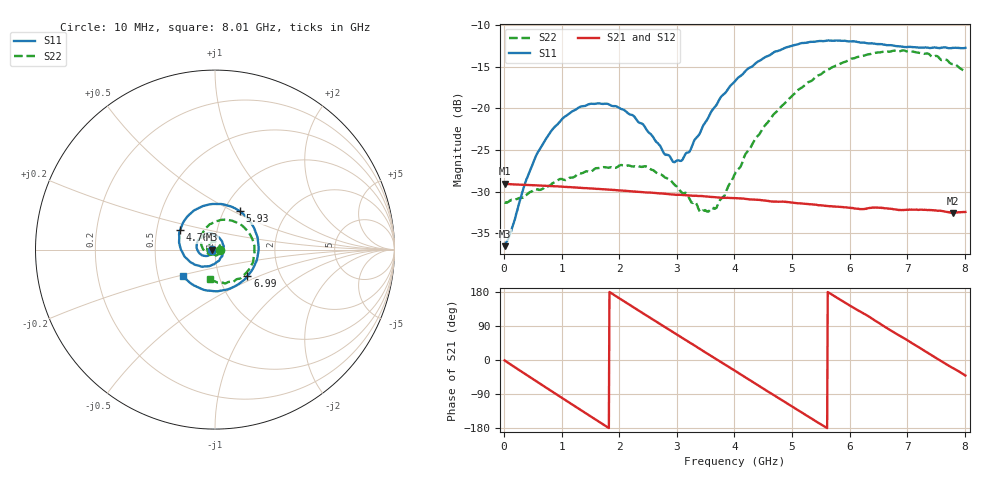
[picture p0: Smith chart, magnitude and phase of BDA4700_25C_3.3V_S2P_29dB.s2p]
!Agilent Technologies,E5071B,MY42404982,A.09.10
!Date: Mon Oct 20 18:15:16 2025
!Data & Calibration Information:
!Freq	S11:SOLT2(ON)	S21:SOLT2(ON)	S12:SOLT2(ON)	S22:SOLT2(ON)
# Hz S RI R 50
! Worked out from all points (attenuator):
!   801 points, 10 MHz to 8.01 GHz, reference 50 ohm
!   highest |S21| = -29.05 dB at 20 MHz (marker M1); lowest = -32.6 dB at 7.8 GHz (marker M2)
!   lowest |S11| = -36.5 dB at 10 MHz (marker M3), VSWR 1.03, Z = 48.5 - j0.123 ohm
!   |S11| at or under -10 dB: start of sweep to end of sweep
!   |S22| runs from -32.5 to -13.0 dB; largest |S21 - S12| = 0.00038
!   S11 on the Smith chart (normalised r, x): 10 MHz: 0.97, -0.00; 4.76 GHz: 0.66, +0.15; 5.93 GHz: 1.19, +0.54; 6.99 GHz: 1.36, -0.43; 8.01 GHz: 0.67, -0.21
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1e7  -0.0148 -0.00126  0.0352 -0.000725  0.0352 -0.000801  0.0272 -0.000793
2e7  -0.0152 -0.00199  0.0352 -0.00132  0.0352 -0.00144  0.0271 -0.00111
5.9e8  -0.042 -0.0353  0.0178 -0.0296  0.0178 -0.0295  0.0139 -0.0295
1e9  -0.0822 -0.0243  -0.00551 -0.0334  -0.00552 -0.0334  -0.0146 -0.0348
1.35e9  -0.1024 0.0116  -0.023 -0.0241  -0.023 -0.0241  -0.0364 -0.0182
2.07e9  -0.046 0.087  -0.0294 0.0129  -0.0293 0.0129  -0.0309 0.0332
2.68e9  0.0378 0.0483  -0.00406 0.0307  -0.00411 0.0306  0.0127 0.0384
2.93e9  0.0475 0.00681  0.00845 0.0292  0.00849 0.0291  0.0249 0.0256
3.06e9  0.0454 -0.0167  0.0145 0.0266  0.0142 0.0266  0.0279 0.0156
3.43e9  0.00301 -0.0752  0.0267 0.0132  0.0267 0.0133  0.0202 -0.0127
3.69e9  -0.0491 -0.0932  0.0292 0.00094  0.0293 0.000862  0.00162 -0.0253
4.01e9  -0.1237 -0.0776  0.0254 -0.0138  0.0254 -0.0137  -0.0309 -0.0261
4.41e9  -0.1915 0.00402  0.0112 -0.0259  0.0113 -0.026  -0.0683 0.00643
4.76e9  -0.1945 0.1076  -0.00461 -0.0271  -0.00451 -0.0271  -0.0783 0.0591
5.35e9  -0.0624 0.2435  -0.0241 -0.011  -0.0241 -0.0111  -0.0161 0.1465
5.93e9  0.1391 0.2134  -0.0222 0.0126  -0.0222 0.0124  0.114 0.1535
6.35e9  0.2304 0.0865  -0.01 0.0232  -0.00988 0.0231  0.1942 0.0854
6.68e9  0.2366 -0.0412  0.00386 0.0247  0.00389 0.0247  0.2195 0.000927
6.99e9  0.1805 -0.1488  0.0147 0.0198  0.0148 0.0197  0.205 -0.082
7.44e9  0.024 -0.231  0.024 0.00467  0.024 0.0047  0.1165 -0.1676
7.8e9  -0.1164 -0.2  0.0219 -0.00866  0.0219 -0.00879  0.0206 -0.1837
8.01e9  -0.179 -0.1467  0.018 -0.0157  0.018 -0.0155  -0.0298 -0.1635
